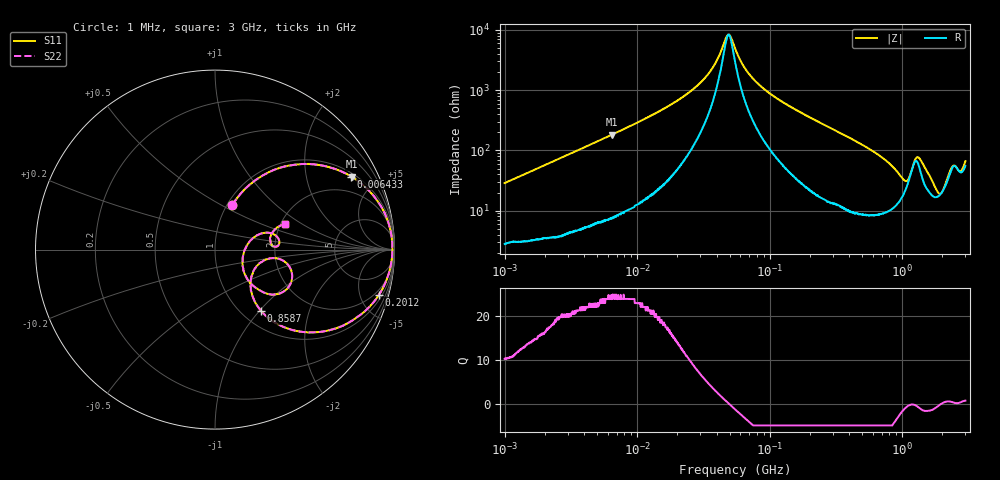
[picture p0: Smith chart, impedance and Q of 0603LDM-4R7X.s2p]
!s-Parameter Generated by FASTRON Sdn. Bhd.
!FASTRON P/N : 0603LDM-4R7X
!Keysight Technologies: E4991B_MY54100416_A.01.15
!Date: Thu Nov 27 16:25:17 2025
!Version  :Rev00  Thu Nov 27 16:25:17 2025
!Data & Calibration Information:
!Freq  S11  S21  S12  S22
!PortZ  Port1:50+j0  Port2:50+j0
!When reading reference impedance value at option line is always used.
! Remarks : This data is being provided solely for informational purposes.
# Hz S dB R 50
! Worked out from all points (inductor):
!   1601 points, 1 MHz to 3 GHz, reference 50 ohm
!   read as one part in series: L = 4.52 uH near 1.041 MHz
!   highest Q = 23.9 at 6.466 MHz (marker M1), where L = 4.5 uH
!   self-resonance near 49.05 MHz
!   S11 on the Smith chart (normalised r, x): 1 MHz: 1.06, +0.57; 6.433 MHz: 1.16, +3.64; 201.2 MHz: 1.44, -7.06; 858.7 MHz: 1.22, -1.02; 3 GHz: 2.10, +0.73
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1000000  -11.40 68.9  -0.56 -15.5  -0.56 -15.5  -11.40 68.9
3804036  -2.92 41.8  -3.51 -45.6  -3.51 -45.6  -2.92 41.8
6433254  -1.30 28.2  -6.50 -59.4  -6.50 -59.4  -1.30 28.2
6465526  -1.28 28.1  -6.53 -59.5  -6.53 -59.5  -1.28 28.1
1.447069e7  -0.32 12.7  -13.20 -74.4  -13.20 -74.4  -0.32 12.7
3.142935e7  -0.12 3.8  -23.50 -76.7  -23.50 -76.7  -0.12 3.8
3.858661e7  -0.10 2.0  -28.80 -69.8  -28.80 -69.8  -0.10 2.0
4.833154e7  -0.10 0.1  -38.40 -9.9  -38.40 -9.9  -0.10 0.1
5.504702e7  -0.10 -0.9  -33.80 53.2  -33.80 53.2  -0.10 -0.9
6.525633e7  -0.11 -2.4  -27.30 71.1  -27.30 71.1  -0.11 -2.4
8.29729e7  -0.14 -4.5  -22.00 76.3  -22.00 76.3  -0.14 -4.5
2.011837e8  -0.47 -15.5  -11.40 71.0  -11.40 71.0  -0.47 -15.5
2.083556e8  -0.50 -16.1  -11.10 70.4  -11.10 70.4  -0.50 -16.1
4.902556e8  -2.37 -36.7  -4.45 49.4  -4.45 49.4  -2.37 -36.7
7.925923e8  -6.15 -51.7  -1.99 29.1  -1.99 29.1  -6.15 -51.7
8.586597e8  -7.38 -53.1  -1.75 24.7  -1.75 24.7  -7.38 -53.1
1.080907e9  -12.20 -28.7  -2.02 8.6  -2.02 8.6  -12.20 -28.7
1.206698e9  -8.90 -8.2  -3.79 4.5  -3.79 4.5  -8.90 -8.2
1.381259e9  -6.93 -30.8  -3.67 20.6  -3.67 20.6  -6.93 -30.8
1.931433e9  -15.90 -11.9  -1.47 2.2  -1.47 2.2  -15.90 -11.9
2.359433e9  -9.24 13.5  -3.49 -6.9  -3.49 -6.9  -9.24 13.5
3e9  -7.65 20.2  -4.05 -13.2  -4.05 -13.2  -7.65 20.2
